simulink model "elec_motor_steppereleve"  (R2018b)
settings: Solver=VariableStepAuto  StartTime=0.0  StopTime=2  FixedStep=0.001  MaxStep=0.001  RelTol=1e-3  EnableMultiTasking=on
libraries: fl_lib x27, nesl_utility x6, elec_lib x2, simulink x1

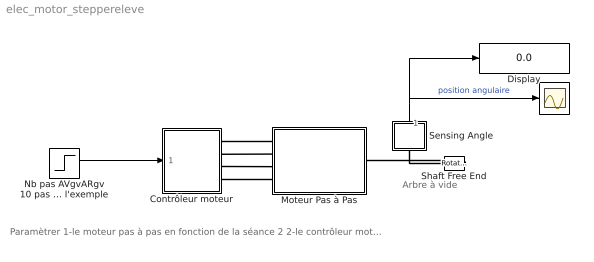
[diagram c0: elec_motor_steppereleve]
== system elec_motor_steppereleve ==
  note: Arbre à vide
  note: Paramètrer 1-le moteur pas à pas en fonction de la séance 2 2-le contrôleur moteur (f<1000Hz)
  " " : Scope
  Contrôleur moteur : Subsystem  mask{f=0}
      mask prompts: f "Fréquence de pilotage (Hz)"
  Display : Display
  Moteur Pas à Pas : Subsystem  mask{R=0, T=0, I=0, pas=0}
      mask prompts: R "Résistance (Ohms)"; T "Couple (Nm)"; I "Intensité (A)"; pas "Pas (°)"
  Nb pas AVgvARgv 10 pas dans l'exemple : Step  Before=10  After=0  SampleTime=0
  Sensing Angle : Subsystem
  Shaft Free End : fl_lib/Mechanical/Rotational Elements/Rotational Free End  w_specify=off  w_priority=None  w=0 rad/s  w_nominal_specify=off  w_nominal_unit=rad/s  w_nominal_value=1
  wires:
  Nb pas AVgvARgv 10 pas dans l'exemple/1 -> Contrôleur moteur/1(In1)
  Sensing Angle/1(theta) -> Display/1, " "/1  "position angulaire"
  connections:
  Contrôleur moteur/RConn1 -- Moteur Pas à Pas/LConn1
  Moteur Pas à Pas/LConn2 -- Contrôleur moteur/RConn2
  Contrôleur moteur/RConn3 -- Moteur Pas à Pas/LConn3
  Contrôleur moteur/RConn4 -- Moteur Pas à Pas/LConn4
  Shaft Free End/LConn1 -- Moteur Pas à Pas/RConn1 -- Sensing Angle/LConn1

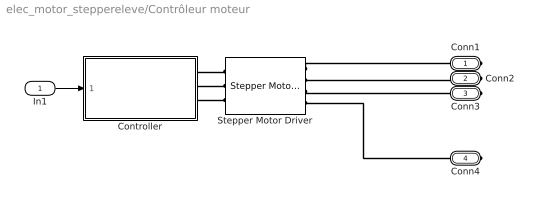
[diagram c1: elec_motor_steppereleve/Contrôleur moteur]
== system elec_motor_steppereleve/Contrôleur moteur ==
  In1 : Inport
  Controller : Subsystem  VariantControlMode=Label  Variant=on  LabelModeActiveChoice=Position
  Stepper Motor Driver : elec_lib/Actuators & Drivers/Drivers/Stepper Motor Driver  step_or_av=1  step_rate_per_volt=10 Hz/V  Venable=2.5 V  Vreverse=2.5 V  Vm=5 V  half_stepping=0
  Conn1 : PMIOPort  Side=Right
  Conn2 : PMIOPort  Port=2  Side=Right
  Conn3 : PMIOPort  Port=3  Side=Right
  Conn4 : PMIOPort  Port=4  Side=Right
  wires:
  In1/1 -> Controller/1(Ref)
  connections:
  Controller/RConn2 -- Stepper Motor Driver/LConn2
  Controller/RConn1 -- Stepper Motor Driver/LConn1
  Stepper Motor Driver/RConn1 -- Conn1/RConn1
  Controller/RConn3 -- Stepper Motor Driver/LConn3
  Stepper Motor Driver/RConn4 -- Conn4/RConn1
  Stepper Motor Driver/RConn3 -- Conn3/RConn1
  Conn2/RConn1 -- Stepper Motor Driver/RConn2

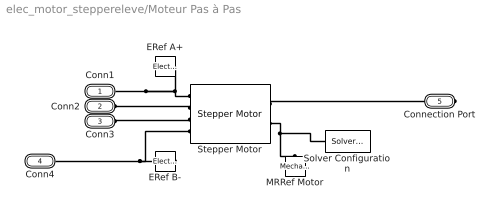
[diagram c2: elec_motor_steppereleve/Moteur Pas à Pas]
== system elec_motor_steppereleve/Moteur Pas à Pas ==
  ERef A+ : fl_lib/Electrical/Electrical Elements/Electrical Reference
  ERef B- : fl_lib/Electrical/Electrical Elements/Electrical Reference
  MRRef Motor : fl_lib/Mechanical/Rotational Elements/Mechanical Rotational Reference
  Solver Configuration : nesl_utility/Solver Configuration  PhysicalDomain=network_engine_domain  SubClassName=solver  LeftPortType=input  RightPortType=generic  Tones=[]  Harmonics=[]  SimulateNoise=off  Profile=off  UseLocalSampling=off  EnableSwitchedLinearOptims=on  FrequencyDomain=off  UseCCode=off  RelTol=0.001  AbsTol=1e-06  MinStep=1e-09  ToWorkspace=off  RevertToSquareIcSolve=off  NumHomotopyIterations=100  PhasorMode=off  PhasorModeNumHarmonics=1  DoDC=off  ResidualTolerance=1e-9  UseLocalSolver=off  LocalSolverChoice=NE_BACKWARD_EULER_ADVANCER  LocalSolverSampleTime=.001  DoFixedCost=off  MaxNonlinIter=3  MaxModeIter=2  LinearAlgebra=auto  EquationFormulation=NE_TIME_EF  DelaysMemoryBudget=1024  AutomaticFiltering=on  FilteringTimeConstant=0.001  PartitionStorageMethod=AS_NEEDED  PartitionMemoryBudget=1024
  Stepper Motor : elec_lib/Actuators & Drivers/Rotational Actuators/Stepper Motor  step_or_av=1  w_vec=[ 0 1000 3e+3 ] rpm  T_vec=[ 2 2 1 ] N*m  assert_if_slipping=0  J_total=1e-4 kg*m^2  max_step_rate=10 Hz  Ra=R Ohm  La=0.0015 H  Km=T/I N*m/A  Td=0 N*m  Rm=Inf Ohm  Step=pas deg  J=4.5e-05 kg*m^2  B=1e-02 N*m/(rad/s)  speed0=0 rpm  theta0=0 deg  alpha=[ 0.00393 0.00393 ] 1/K  Tmeas=25 degC  T_vec2=[ 1.7 1.7 0.85 ] N*m  Tmeas2=125 degC  half_stepping=0  thermal_masses=[ 100 100 ] J/K  initial_temperatures=[ 25 25 ] degC  rotor_thermal_mass=50 J/K  rotor_initial_temperature=25 degC  Rm_percent_rotor=90
  Conn1 : PMIOPort  Side=Left
  Conn2 : PMIOPort  Port=2  Side=Left
  Conn3 : PMIOPort  Port=3  Side=Left
  Conn4 : PMIOPort  Port=4  Side=Left
  Connection Port : PMIOPort  Port=5  Side=Right
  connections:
  Stepper Motor/RConn2 -- Solver Configuration/RConn1 -- MRRef Motor/LConn1
  Stepper Motor/LConn1 -- Conn1/RConn1 -- ERef A+/LConn1
  Stepper Motor/RConn1 -- Connection Port/RConn1
  ERef B-/LConn1 -- Stepper Motor/LConn4 -- Conn4/RConn1
  Conn3/RConn1 -- Stepper Motor/LConn3
  Stepper Motor/LConn2 -- Conn2/RConn1

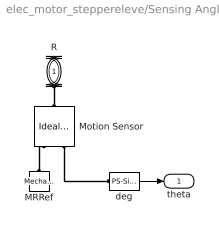
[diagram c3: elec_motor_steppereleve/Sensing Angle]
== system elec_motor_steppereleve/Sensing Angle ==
  MRRef : fl_lib/Mechanical/Rotational Elements/Mechanical Rotational Reference
  Motion Sensor : fl_lib/Mechanical/Mechanical Sensors/Ideal Rotational Motion Sensor  offset=0 rad
  deg : nesl_utility/PS-Simulink Converter  PhysicalDomain=network_engine_domain  SubClassName=ps_output  LeftPortType=input  RightPortType=output  PseudoPeriodic=off  Frequencies=[]  Unit=deg  AffineConversion=off
  R : PMIOPort  Side=Left
  theta : Outport
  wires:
  deg/1 -> theta/1
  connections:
  R/RConn1 -- Motion Sensor/LConn1
  Motion Sensor/RConn3 -- deg/LConn1
  MRRef/LConn1 -- Motion Sensor/RConn1

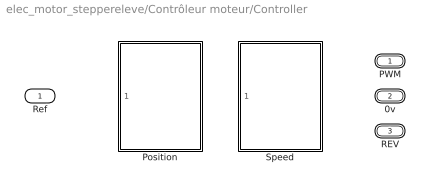
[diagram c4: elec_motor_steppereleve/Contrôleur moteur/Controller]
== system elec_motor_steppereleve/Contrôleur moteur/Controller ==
  Ref : Inport
  Position : Subsystem  VariantControl=Position
  Speed : Subsystem  VariantControl=Speed
  PWM : PMIOPort  Side=Right
  0v : PMIOPort  Port=2  Side=Right
  REV : PMIOPort  Port=3  Side=Right

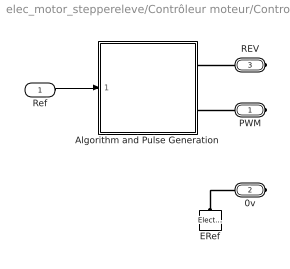
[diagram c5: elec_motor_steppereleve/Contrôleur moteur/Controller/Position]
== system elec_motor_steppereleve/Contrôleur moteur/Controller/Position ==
  Ref : Inport
  Algorithm and Pulse Generation : Subsystem
  ERef : fl_lib/Electrical/Electrical Elements/Electrical Reference
  PWM : PMIOPort  Side=Right
  0v : PMIOPort  Port=2  Side=Right
  REV : PMIOPort  Port=3  Side=Right
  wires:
  Ref/1 -> Algorithm and Pulse Generation/1(Reference)
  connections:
  Algorithm and Pulse Generation/RConn2 -- PWM/RConn1
  Algorithm and Pulse Generation/RConn1 -- REV/RConn1
  ERef/LConn1 -- 0v/RConn1

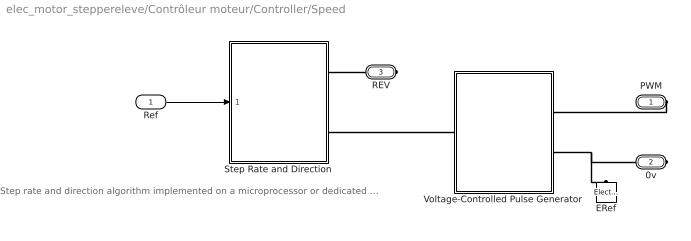
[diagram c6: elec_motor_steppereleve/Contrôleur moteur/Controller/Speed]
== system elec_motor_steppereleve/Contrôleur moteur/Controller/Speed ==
  note: Step rate and direction algorithm implemented on a microprocessor or dedicated discrete chip
  Ref : Inport
  ERef : fl_lib/Electrical/Electrical Elements/Electrical Reference
  Step Rate and Direction : Subsystem
  Voltage-Controlled Pulse Generator : Subsystem
  PWM : PMIOPort  Side=Right
  0v : PMIOPort  Port=2  Side=Right
  REV : PMIOPort  Port=3  Side=Right
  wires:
  Ref/1 -> Step Rate and Direction/1(Reference)
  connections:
  PWM/RConn1 -- Voltage-Controlled Pulse Generator/RConn1
  Voltage-Controlled Pulse Generator/RConn2 -- 0v/RConn1 -- ERef/LConn1
  Step Rate and Direction/RConn1 -- REV/RConn1
  Step Rate and Direction/RConn2 -- Voltage-Controlled Pulse Generator/LConn1

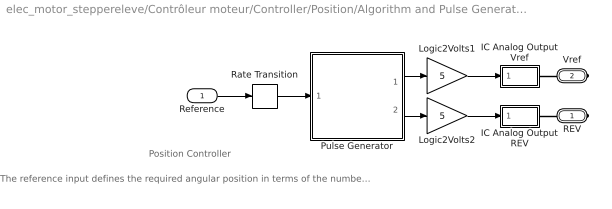
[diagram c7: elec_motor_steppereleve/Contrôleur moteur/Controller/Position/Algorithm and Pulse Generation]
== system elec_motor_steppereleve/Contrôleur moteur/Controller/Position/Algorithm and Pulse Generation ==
  note: The reference input defines the required angular position in terms of the number steps. For this stepper, the step size is 1.8 degrees. Hence a demand of 10 steps results in an angle change of 18 degrees. The step rate is set by the Pulse Generator's Pulse rate mask parameter.
  note: Position Controller
  Reference : Inport
  IC Analog Output REV : Subsystem
  IC Analog Output Vref : Subsystem
  Logic2Volts1 : Gain  Gain=5
  Logic2Volts2 : Gain  Gain=5
  Pulse Generator : Subsystem  mask{f=f}
      mask prompts: f "Pulse rate"
  Rate Transition : RateTransition  Deterministic=off
  REV : PMIOPort  Side=Right
  Vref : PMIOPort  Port=2  Side=Right
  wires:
  Logic2Volts1/1 -> IC Analog Output Vref/1(SL)
  Pulse Generator/1(Pulse train) -> Logic2Volts1/1
  Reference/1 -> Rate Transition/1
  Logic2Volts2/1 -> IC Analog Output REV/1(SL)
  Pulse Generator/2(Pulse direction) -> Logic2Volts2/1
  Rate Transition/1 -> Pulse Generator/1(Pulse  demand)
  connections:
  Vref/RConn1 -- IC Analog Output Vref/RConn1
  REV/RConn1 -- IC Analog Output REV/RConn1

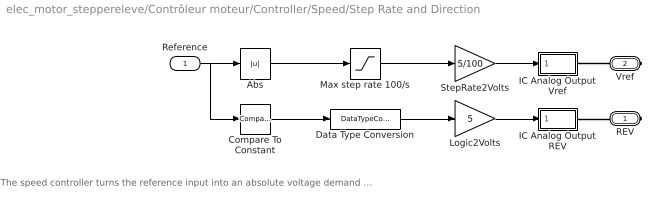
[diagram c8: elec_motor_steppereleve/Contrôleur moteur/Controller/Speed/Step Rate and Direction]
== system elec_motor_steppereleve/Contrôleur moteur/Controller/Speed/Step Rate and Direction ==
  note: The speed controller turns the reference input into an absolute voltage demand for the voltage-controlled pulse generator and sets the reverse flag signal to +5 volts when the speed demand is negative.
  Reference : Inport
  Abs : Abs
  Compare To Constant : simulink/Logic and Bit Operations/Compare To Constant  relop=<  const=0  OutDataTypeStr=uint8  ZeroCross=off
  Data Type Conversion : DataTypeConversion
  IC Analog Output REV : Subsystem
  IC Analog Output Vref : Subsystem
  Logic2Volts : Gain  Gain=5
  Max step rate 100/s : Saturate  UpperLimit=100  LowerLimit=0
  StepRate2Volts : Gain  Gain=5/100
  REV : PMIOPort  Side=Right
  Vref : PMIOPort  Port=2  Side=Right
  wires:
  StepRate2Volts/1 -> IC Analog Output Vref/1(SL)
  Max step rate 100/s/1 -> StepRate2Volts/1
  Data Type Conversion/1 -> Logic2Volts/1
  Compare To Constant/1 -> Data Type Conversion/1
  Reference/1 -> Compare To Constant/1, Abs/1
  Abs/1 -> Max step rate 100/s/1
  Logic2Volts/1 -> IC Analog Output REV/1(SL)
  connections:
  REV/RConn1 -- IC Analog Output REV/RConn1
  Vref/RConn1 -- IC Analog Output Vref/RConn1

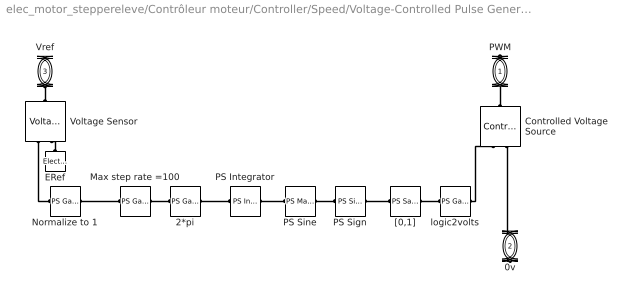
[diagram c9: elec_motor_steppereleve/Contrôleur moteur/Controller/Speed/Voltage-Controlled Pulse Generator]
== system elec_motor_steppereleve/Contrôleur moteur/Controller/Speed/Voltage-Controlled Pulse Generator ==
  2*pi : fl_lib/Physical Signals/Functions/PS Gain  gain=-2*pi
  Controlled Voltage Source : fl_lib/Electrical/Electrical Sources/Controlled Voltage Source
  ERef : fl_lib/Electrical/Electrical Elements/Electrical Reference
  Max step rate =100 : fl_lib/Physical Signals/Functions/PS Gain  gain=100
  Normalize to 1 : fl_lib/Physical Signals/Functions/PS Gain  gain=1/5
  PS Integrator : fl_lib/Physical Signals/Linear Operators/PS Integrator  x0=0
  PS Sign : fl_lib/Physical Signals/Nonlinear Operators/PS Sign
  PS Sine : fl_lib/Physical Signals/Functions/PS Math Function  fcn_choice=1
  Voltage Sensor : fl_lib/Electrical/Electrical Sensors/Voltage Sensor
  "[0,1]" : fl_lib/Physical Signals/Nonlinear Operators/PS Saturation  upper_limit=1  lower_limit=0
  logic2volts : fl_lib/Physical Signals/Functions/PS Gain  gain=5
  PWM : PMIOPort  Side=Right
  0v : PMIOPort  Port=2  Side=Right
  Vref : PMIOPort  Port=3  Side=Left
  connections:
  PWM/RConn1 -- Controlled Voltage Source/LConn1
  Controlled Voltage Source/RConn2 -- 0v/RConn1
  Vref/RConn1 -- Voltage Sensor/LConn1
  ERef/LConn1 -- Voltage Sensor/RConn2
  Voltage Sensor/RConn1 -- Normalize to 1/LConn1
  Max step rate =100/LConn1 -- Normalize to 1/RConn1
  Max step rate =100/RConn1 -- 2*pi/LConn1
  2*pi/RConn1 -- PS Integrator/LConn1
  PS Integrator/RConn1 -- PS Sine/LConn1
  PS Sign/LConn1 -- PS Sine/RConn1
  "[0,1]"/LConn1 -- PS Sign/RConn1
  "[0,1]"/RConn1 -- logic2volts/LConn1
  logic2volts/RConn1 -- Controlled Voltage Source/RConn1

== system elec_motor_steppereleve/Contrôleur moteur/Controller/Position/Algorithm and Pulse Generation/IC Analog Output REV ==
  SL : Inport
  Controlled Voltage Source : fl_lib/Electrical/Electrical Sources/Controlled Voltage Source
  ERef : fl_lib/Electrical/Electrical Elements/Electrical Reference
  Simulink-PS Converter : nesl_utility/Simulink-PS Converter  PhysicalDomain=network_engine_domain  SubClassName=ps_input  LeftPortType=input  RightPortType=output  PseudoPeriodic=off  Frequencies=[]  NoiseDistribution=none  NoiseParameters=[]  Unit=V  AffineConversion=off  FilteringAndDerivatives=zero  SimscapeFilterOrder=1  InputFilterTimeConstant=.001  UdotUserProvided=0
  V : PMIOPort  Side=Right
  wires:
  SL/1 -> Simulink-PS Converter/1
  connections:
  ERef/LConn1 -- Controlled Voltage Source/RConn2
  V/RConn1 -- Controlled Voltage Source/LConn1
  Simulink-PS Converter/RConn1 -- Controlled Voltage Source/RConn1

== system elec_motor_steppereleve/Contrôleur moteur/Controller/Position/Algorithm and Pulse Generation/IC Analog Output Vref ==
  SL : Inport
  Controlled Voltage Source : fl_lib/Electrical/Electrical Sources/Controlled Voltage Source
  ERef : fl_lib/Electrical/Electrical Elements/Electrical Reference
  Simulink-PS Converter : nesl_utility/Simulink-PS Converter  PhysicalDomain=network_engine_domain  SubClassName=ps_input  LeftPortType=input  RightPortType=output  PseudoPeriodic=off  Frequencies=[]  NoiseDistribution=none  NoiseParameters=[]  Unit=V  AffineConversion=off  FilteringAndDerivatives=zero  SimscapeFilterOrder=1  InputFilterTimeConstant=.001  UdotUserProvided=0
  V : PMIOPort  Side=Right
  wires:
  SL/1 -> Simulink-PS Converter/1
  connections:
  Simulink-PS Converter/RConn1 -- Controlled Voltage Source/RConn1
  V/RConn1 -- Controlled Voltage Source/LConn1
  ERef/LConn1 -- Controlled Voltage Source/RConn2

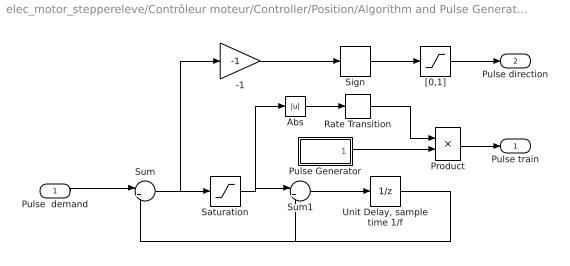
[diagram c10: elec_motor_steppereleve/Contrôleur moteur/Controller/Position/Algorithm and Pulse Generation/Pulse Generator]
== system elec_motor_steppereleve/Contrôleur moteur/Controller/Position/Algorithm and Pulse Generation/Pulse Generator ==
  Pulse  demand : Inport  SampleTime=1/f
  -1 : Gain  Gain=-1
  Abs : Abs
  Product : Product
  Pulse Generator : Subsystem
  Rate Transition : RateTransition  Deterministic=off
  Saturation : Saturate  UpperLimit=1  LowerLimit=-1
  Sign : Signum
  Sum : Sum  Inputs=|+-
  Sum1 : Sum  Inputs=|++
  "Unit Delay, sample time 1/f" : UnitDelay  SampleTime=1/f
  "[0,1]" : Saturate  UpperLimit=1  LowerLimit=0
  Pulse train : Outport
  Pulse direction : Outport  Port=2
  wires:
  "[0,1]"/1 -> Pulse direction/1
  -1/1 -> Sign/1
  "Unit Delay, sample time 1/f"/1 -> Sum/2, Sum1/2
  Pulse  demand/1 -> Sum/1
  Sum/1 -> -1/1, Saturation/1
  Saturation/1 -> Sum1/1, Abs/1
  Sum1/1 -> "Unit Delay, sample time 1/f"/1
  Sign/1 -> "[0,1]"/1
  Product/1 -> Pulse train/1
  Abs/1 -> Rate Transition/1
  Pulse Generator/1(p) -> Product/2
  Rate Transition/1 -> Product/1

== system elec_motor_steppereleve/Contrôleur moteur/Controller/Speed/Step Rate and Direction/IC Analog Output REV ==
  SL : Inport
  Controlled Voltage Source : fl_lib/Electrical/Electrical Sources/Controlled Voltage Source
  ERef : fl_lib/Electrical/Electrical Elements/Electrical Reference
  Simulink-PS Converter : nesl_utility/Simulink-PS Converter  PhysicalDomain=network_engine_domain  SubClassName=ps_input  LeftPortType=input  RightPortType=output  PseudoPeriodic=off  Frequencies=[]  NoiseDistribution=none  NoiseParameters=[]  Unit=V  AffineConversion=off  FilteringAndDerivatives=zero  SimscapeFilterOrder=1  InputFilterTimeConstant=.001  UdotUserProvided=0
  V : PMIOPort  Side=Right
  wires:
  SL/1 -> Simulink-PS Converter/1
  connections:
  Simulink-PS Converter/RConn1 -- Controlled Voltage Source/RConn1
  V/RConn1 -- Controlled Voltage Source/LConn1
  ERef/LConn1 -- Controlled Voltage Source/RConn2

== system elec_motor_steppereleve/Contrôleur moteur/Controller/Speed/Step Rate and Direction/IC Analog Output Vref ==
  SL : Inport
  Controlled Voltage Source : fl_lib/Electrical/Electrical Sources/Controlled Voltage Source
  ERef : fl_lib/Electrical/Electrical Elements/Electrical Reference
  Simulink-PS Converter : nesl_utility/Simulink-PS Converter  PhysicalDomain=network_engine_domain  SubClassName=ps_input  LeftPortType=input  RightPortType=output  PseudoPeriodic=off  Frequencies=[]  NoiseDistribution=none  NoiseParameters=[]  Unit=V  AffineConversion=off  FilteringAndDerivatives=zero  SimscapeFilterOrder=1  InputFilterTimeConstant=.001  UdotUserProvided=0
  V : PMIOPort  Side=Right
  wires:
  SL/1 -> Simulink-PS Converter/1
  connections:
  ERef/LConn1 -- Controlled Voltage Source/RConn2
  V/RConn1 -- Controlled Voltage Source/LConn1
  Simulink-PS Converter/RConn1 -- Controlled Voltage Source/RConn1

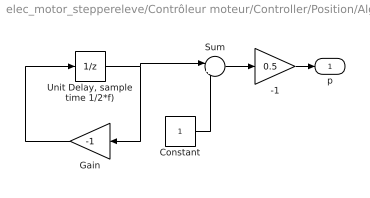
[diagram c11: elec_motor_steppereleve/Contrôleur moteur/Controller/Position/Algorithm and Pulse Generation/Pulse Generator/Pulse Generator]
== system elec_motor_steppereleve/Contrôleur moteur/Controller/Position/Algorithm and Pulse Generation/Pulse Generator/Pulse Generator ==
  -1 : Gain  Gain=0.5
  Constant : Constant  SampleTime=1/(2*f)
  Gain : Gain  Gain=-1
  Sum : Sum  Inputs=|++
  "Unit Delay, sample time 1/2*f)" : UnitDelay  InitialCondition=-1  SampleTime=1/(2*f)
  p : Outport
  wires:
  "Unit Delay, sample time 1/2*f)"/1 -> Gain/1, Sum/1
  Gain/1 -> "Unit Delay, sample time 1/2*f)"/1
  Constant/1 -> Sum/2
  Sum/1 -> -1/1
  -1/1 -> p/1
